|Texas Instruments Incorporated
| Programmable PCM Codec With Microphone Amps & Speaker Driver
| Marketing part#   Digital Voltage Range   Package-type   #pins
| TLV320A1110PBSRG4   2.7-3.3V   TQFP   32
| TLV320AIC1110PBS   2.7-3.3V   TQFP   32
| TLV320AIC1110PBSG4  2.7-3.3V   TQFP   32
| TLV320AIC1110PBSR   2.7-3.3V   TQFP   32
| TLV320AIC1110GQER   2.7-3.3V   BGA MICROSTAR JUNIOR   80
| TLV320AIC1110ZQER   2.7-3.3V   BGA MICROSTAR JUNIOR   80
[IBIS Ver]   3.2
[File name]   tlv320aic1110.ibs
|SIMDE Ver   V2.1 - 201006 - RHL4 - Build 390
[File Rev]   1.1
[Date]   10/06/2010
[Source]
| Texas Instruments Incorporated.
| Analog-eLab Design Center, HPA
| 12500 TI Blvd
| Dallas, TX -75243
| e-mail: elab_ibis@list.ti.com
| -Model generated from simulations in TISPICE
[Notes]   Revision History:
| Rev 1.0: 9/20/2010
| - Initial version of the model
| - Model generated from simulations in TISPICE
| - Model matched to SPICE simulation
| - C_comp although listed in numerical order of value are
|   obtained from varying PVT conditions. For PVT conditions for
|   each specific value refer the buffer description under
|   respective [Model]. IBIS model user is responsible for using
|   appropriate C_comp to simulate for Signal Integrity.
| Rev 1.1: 10/06/2010
| - io_open_drain_sda model VT table changed as per the review comments
[Disclaimer]
| This model is designed as an aid for customers of Texas Instruments.
| TI and its licensors and suppliers make no warranties, either expressed
| or implied, with respect to this  model, including the warranties of
| merchantability or fitness for a particular purpose. The model is
| provided solely on an "as is" basis. The entire risk as to its quality
| and performance is with the customer.
[Copyright]
 (C) Copyright 2010 Texas Instruments Incorporated.All rights reserved.
|   TLV320A1110PBSRG4/TLV320AIC1110PBS
[Component]   TLV320APBS
[Manufacturer]   TI
[Package]   |32 TQFP -  PBS package
|   typ   min   max
R_pkg   0.07184   0.06082   0.08808
L_pkg   2.28640nH   2.01650nH   2.68526nH
C_pkg   0.41135pF   0.38899pF   0.44791pF
[Pin]  signal_name   model_name   R_pin   L_pin   C_pin
1   MBIAS   TERM   0.08808   2.68526nH  0.41328pF
2   MIC1P   TERM   0.08391   2.54706nH  0.44791pF
3   MIC1N   TERM   0.07761   2.36771nH  0.42261pF
4   MIC2P   TERM   0.07618   2.30817nH  0.40996pF
5   MIC2N   TERM   0.07392   2.26536nH  0.40736pF
6   REXT   TERM   0.07368   2.29403nH  0.41316pF
7   MUXIN   TERM   0.07406   2.35917nH  0.43037pF
8   AVSS   GND   0.07533   2.44246nH  0.39927pF
9   MUXOUT1   TERM   0.07051   2.35058nH  0.39571pF
10   MUXOUT2   TERM   0.06517   2.18984nH  0.42182pF
11   SDA   io_opendrain_sda   0.06308   2.09272nH  0.40201pF
12   SCL   input_buffer   0.06082   2.01650nH  0.38966pF
13   DVDD   POWER   0.06336   2.06557nH  0.39394pF
14   DVSS   GND   0.06443   2.11869nH  0.40617pF
15   PCMI   input_buffer   0.06617   2.20906nH  0.42378pF
16   PCMO   tribuf_pcmo   0.07066   2.35247nH  0.39516pF
17   PCMCLK   input_pcmclk   0.07585   2.45373nH  0.39944pF
18   PCMSYN   input_buffer   0.07430   2.36520nH  0.42894pF
19   BUZZCON   tribuf_buzzcon   0.07499   2.32159nH  0.41275pF
20   PWRUPSEL   input_buffer   0.07407   2.26942nH  0.40286pF
21   _RESET   input_buffer   0.07381   2.26355nH  0.40434pF
22   MCLK   input_buffer   0.07436   2.30635nH  0.41540pF
23   VSS   GND   0.07577   2.38981nH  0.42966pF
24   PLLVSS   GND   0.08248   2.57901nH  0.40523pF
25   PLLVDD   POWER   0.07827   2.49816nH  0.40632pF
26   EARVSS   GND   0.07087   2.29522nH  0.43093pF
27   EAR1ON   TERM   0.06675   2.15760nH  0.40779pF
28   EARVDD   POWER   0.06793   2.14724nH  0.39773pF
29   EAR1OP   TERM   0.06150   2.02275nH  0.38899pF
30   EARVSS   GND   0.06028   2.03156nH  0.39750pF
31   EAR2O   TERM   0.06102   2.10259nH  0.41646pF
32   AVDD   POWER   0.06936   2.32089nH  0.39339pF
|   TLV320AIC1110GQER
[Component]   TLV320AIC1110GQER
[Manufacturer]   TI
[Package]   |80 BGA MICROSTAR JUNIOR - GQE package
|   typ   min   max
R_pkg   0.08490   0.06932   0.10116
L_pkg   1.58174nH   1.29375nH   1.88655nH
C_pkg   0.25756pF   0.23973pF   0.27588pF
[Pin]  signal_name   model_name   R_pin   L_pin   C_pin
A1   AVDD   POWER   0.09674  1.81151nH  0.23866pF
A2   EAR2O   TERM   0.08106  1.51327nH  0.25868pF
A3   EARVSS   GND   0.07517  1.40385nH  0.24777pF
A4   EAR1OP   TERM   0.07128  1.33092nH  0.24248pF
A5   EARVDD   POWER   0.07503  1.39865nH  0.24630pF
A6   EAR1ON   TERM   0.07460  1.38924nH  0.24697pF
A7   EARVSS   GND   0.08068  1.50050nH  0.25675pF
A8   PLLVDD   POWER   0.09065  1.68435nH  0.27183pF
A9   PLLVSS   GND   0.10018  1.86705nH  0.24341pF
B1   MBIAS   TERM   0.10116  1.88655nH  0.27588pF
B2   NC   NC   0.00000  0.00000nH  0.00000pF
B3   NC   NC   0.00000  0.00000nH  0.00000pF
B4   NC   NC   0.00000  0.00000nH  0.00000pF
B5   NC   NC   0.00000  0.00000nH  0.00000pF
B6   NC   NC   0.00000  0.00000nH  0.00000pF
B7   NC   NC   0.00000  0.00000nH  0.00000pF
B8   NC   NC   0.00000  0.00000nH  0.00000pF
B9   VSS   GND   0.09705  1.80167nH  0.27101pF
C1   MIC1P   TERM   0.09467  1.76610nH  0.27374pF
C2   NC   NC   0.00000  0.00000nH  0.00000pF
C4   NC   NC   0.00000  0.00000nH  0.00000pF
C5   NC   NC   0.00000  0.00000nH  0.00000pF
C6   NC   NC   0.00000  0.00000nH  0.00000pF
C7   NC   NC   0.00000  0.00000nH  0.00000pF
C8   NC   NC   0.00000  0.00000nH  0.00000pF
C9   MCLK   input_buffer   0.09113  1.69175nH  0.26699pF
D1   MIC1N   TERM   0.08667  1.61834nH  0.26258pF
D2   NC   NC   0.00000  0.00000nH  0.00000pF
D3   NC   NC   0.00000  0.00000nH  0.00000pF
D4   NC   NC   0.00000  0.00000nH  0.00000pF
D5   NC   NC   0.00000  0.00000nH  0.00000pF
D6   NC   NC   0.00000  0.00000nH  0.00000pF
D7   NC   NC   0.00000  0.00000nH  0.00000pF
D8   NC   NC   0.00000  0.00000nH  0.00000pF
D9   _RESET   input_buffer   0.08532  1.58372nH  0.25858pF
E1   MIC2P   TERM   0.08374  1.56425nH  0.25743pF
E2   NC   NC   0.00000  0.00000nH  0.00000pF
E3   NC   NC   0.00000  0.00000nH  0.00000pF
E4   NC   NC   0.00000  0.00000nH  0.00000pF
E5   NC   NC   0.00000  0.00000nH  0.00000pF
E6   NC   NC   0.00000  0.00000nH  0.00000pF
E7   NC   NC   0.00000  0.00000nH  0.00000pF
E8   NC   NC   0.00000  0.00000nH  0.00000pF
E9   PWRUPSEL   input_buffer   0.08338  1.54785nH  0.25370pF
F1   MIC2N   TERM   0.08482  1.58422nH  0.25973pF
F2   NC   NC   0.00000  0.00000nH  0.00000pF
F3   NC   NC   0.00000  0.00000nH  0.00000pF
F4   NC   NC   0.00000  0.00000nH  0.00000pF
F5   NC   NC   0.00000  0.00000nH  0.00000pF
F6   NC   NC   0.00000  0.00000nH  0.00000pF
F7   NC   NC   0.00000  0.00000nH  0.00000pF
F8   NC   NC   0.00000  0.00000nH  0.00000pF
F9   BUZZCON   tribuf_buzzcon   0.08449  1.56834nH  0.25426pF
G1   REXT   TERM   0.08858  1.65365nH  0.26206pF
G2   NC   NC   0.00000  0.00000nH  0.00000pF
G3   NC   NC   0.00000  0.00000nH  0.00000pF
G4   NC   NC   0.00000  0.00000nH  0.00000pF
G5   NC   NC   0.00000  0.00000nH  0.00000pF
G6   NC   NC   0.00000  0.00000nH  0.00000pF
G7   NC   NC   0.00000  0.00000nH  0.00000pF
G8   NC   NC   0.00000  0.00000nH  0.00000pF
G9   PCMSYN   input_buffer   0.08501  1.57820nH  0.25589pF
H1   MUXIN   TERM   0.09293  1.73427nH  0.27014pF
H2   NC   NC   0.00000  0.00000nH  0.00000pF
H3   NC   NC   0.00000  0.00000nH  0.00000pF
H4   NC   NC   0.00000  0.00000nH  0.00000pF
H5   NC   NC   0.00000  0.00000nH  0.00000pF
H6   NC   NC   0.00000  0.00000nH  0.00000pF
H7   NC   NC   0.00000  0.00000nH  0.00000pF
H8   NC   NC   0.00000  0.00000nH  0.00000pF
H9   PCMCLK   input_pcmclk   0.08868  1.64665nH  0.26211pF
J1   AVSS   GND   0.09974  1.86771nH  0.24131pF
J2   MUXOUT1   TERM   0.08328  1.55465nH  0.25850pF
J3   MUXOUT2   TERM   0.07537  1.40740nH  0.24832pF
J4   SDA   io_opendrain_sda   0.07152  1.33564nH  0.24231pF
J5   SCL   input_buffer   0.06932  1.29375nH  0.23973pF
J6   DVDD   POWER   0.07563  1.40832nH  0.24969pF
J7   DVSS   GND   0.08301  1.54355nH  0.26144pF
J8   PCMI   input_buffer   0.09030  1.67757nH  0.27218pF
J9   PCMO   tribuf_pcmo   0.10040  1.87191nH  0.24396pF
|   TLV320AIC1110ZQER
[Component]   TLV320AIC1110ZQER
[Manufacturer]   TI
[Package]   |80 BGA MICROSTAR JUNIOR - ZQE package
|   typ   min   max
R_pkg   0.08490   0.06932   0.10116
L_pkg   1.58174nH   1.29375nH   1.88655nH
C_pkg   0.25756pF   0.23973pF   0.27588pF
[Pin]  signal_name   model_name   R_pin   L_pin   C_pin
A1   AVDD   POWER   0.09674  1.81151nH  0.23866pF
A2   EAR2O   TERM   0.08106  1.51327nH  0.25868pF
A3   EARVSS   GND   0.07517  1.40385nH  0.24777pF
A4   EAR1OP   TERM   0.07128  1.33092nH  0.24248pF
A5   EARVDD   POWER   0.07503  1.39865nH  0.24630pF
A6   EAR1ON   TERM   0.07460  1.38924nH  0.24697pF
A7   EARVSS   GND   0.08068  1.50050nH  0.25675pF
A8   PLLVDD   POWER   0.09065  1.68435nH  0.27183pF
A9   PLLVSS   GND   0.10018  1.86705nH  0.24341pF
B1   MBIAS   TERM   0.10116  1.88655nH  0.27588pF
B2   NC   NC   0.00000  0.00000nH  0.00000pF
B3   NC   NC   0.00000  0.00000nH  0.00000pF
B4   NC   NC   0.00000  0.00000nH  0.00000pF
B5   NC   NC   0.00000  0.00000nH  0.00000pF
B6   NC   NC   0.00000  0.00000nH  0.00000pF
B7   NC   NC   0.00000  0.00000nH  0.00000pF
B8   NC   NC   0.00000  0.00000nH  0.00000pF
B9   VSS   GND   0.09705  1.80167nH  0.27101pF
C1   MIC1P   TERM   0.09467  1.76610nH  0.27374pF
C2   NC   NC   0.00000  0.00000nH  0.00000pF
C4   NC   NC   0.00000  0.00000nH  0.00000pF
C5   NC   NC   0.00000  0.00000nH  0.00000pF
C6   NC   NC   0.00000  0.00000nH  0.00000pF
C7   NC   NC   0.00000  0.00000nH  0.00000pF
C8   NC   NC   0.00000  0.00000nH  0.00000pF
C9   MCLK   input_buffer   0.09113  1.69175nH  0.26699pF
D1   MIC1N   TERM   0.08667  1.61834nH  0.26258pF
D2   NC   NC   0.00000  0.00000nH  0.00000pF
D3   NC   NC   0.00000  0.00000nH  0.00000pF
D4   NC   NC   0.00000  0.00000nH  0.00000pF
D5   NC   NC   0.00000  0.00000nH  0.00000pF
D6   NC   NC   0.00000  0.00000nH  0.00000pF
D7   NC   NC   0.00000  0.00000nH  0.00000pF
D8   NC   NC   0.00000  0.00000nH  0.00000pF
D9   _RESET   input_buffer   0.08532  1.58372nH  0.25858pF
E1   MIC2P   TERM   0.08374  1.56425nH  0.25743pF
E2   NC   NC   0.00000  0.00000nH  0.00000pF
E3   NC   NC   0.00000  0.00000nH  0.00000pF
E4   NC   NC   0.00000  0.00000nH  0.00000pF
E5   NC   NC   0.00000  0.00000nH  0.00000pF
E6   NC   NC   0.00000  0.00000nH  0.00000pF
E7   NC   NC   0.00000  0.00000nH  0.00000pF
E8   NC   NC   0.00000  0.00000nH  0.00000pF
E9   PWRUPSEL   input_buffer   0.08338  1.54785nH  0.25370pF
F1   MIC2N   TERM   0.08482  1.58422nH  0.25973pF
F2   NC   NC   0.00000  0.00000nH  0.00000pF
F3   NC   NC   0.00000  0.00000nH  0.00000pF
F4   NC   NC   0.00000  0.00000nH  0.00000pF
F5   NC   NC   0.00000  0.00000nH  0.00000pF
F6   NC   NC   0.00000  0.00000nH  0.00000pF
F7   NC   NC   0.00000  0.00000nH  0.00000pF
F8   NC   NC   0.00000  0.00000nH  0.00000pF
F9   BUZZCON   tribuf_buzzcon   0.08449  1.56834nH  0.25426pF
G1   REXT   TERM   0.08858  1.65365nH  0.26206pF
G2   NC   NC   0.00000  0.00000nH  0.00000pF
G3   NC   NC   0.00000  0.00000nH  0.00000pF
G4   NC   NC   0.00000  0.00000nH  0.00000pF
G5   NC   NC   0.00000  0.00000nH  0.00000pF
G6   NC   NC   0.00000  0.00000nH  0.00000pF
G7   NC   NC   0.00000  0.00000nH  0.00000pF
G8   NC   NC   0.00000  0.00000nH  0.00000pF
G9   PCMSYN   input_buffer   0.08501  1.57820nH  0.25589pF
H1   MUXIN   TERM   0.09293  1.73427nH  0.27014pF
H2   NC   NC   0.00000  0.00000nH  0.00000pF
H3   NC   NC   0.00000  0.00000nH  0.00000pF
H4   NC   NC   0.00000  0.00000nH  0.00000pF
H5   NC   NC   0.00000  0.00000nH  0.00000pF
H6   NC   NC   0.00000  0.00000nH  0.00000pF
H7   NC   NC   0.00000  0.00000nH  0.00000pF
H8   NC   NC   0.00000  0.00000nH  0.00000pF
H9   PCMCLK   input_pcmclk   0.08868  1.64665nH  0.26211pF
J1   AVSS   GND   0.09974  1.86771nH  0.24131pF
J2   MUXOUT1   TERM   0.08328  1.55465nH  0.25850pF
J3   MUXOUT2   TERM   0.07537  1.40740nH  0.24832pF
J4   SDA   io_opendrain_sda   0.07152  1.33564nH  0.24231pF
J5   SCL   input_buffer   0.06932  1.29375nH  0.23973pF
J6   DVDD   POWER   0.07563  1.40832nH  0.24969pF
J7   DVSS   GND   0.08301  1.54355nH  0.26144pF
J8   PCMI   input_buffer   0.09030  1.67757nH  0.27218pF
J9   PCMO   tribuf_pcmo   0.10040  1.87191nH  0.24396pF
[Model]  TERM
Model_type Terminator
C_comp   1.0e-20F  1.0e-20F  1.0e-20F
|   typ   min   max
[Voltage Range]   3.0V   2.7V   3.3V
[POWER Clamp Reference]   3.0V   2.7V   3.3V
[GND Clamp Reference]   0V   0V   0V
|Ambient Temperature   25   105   -40
|Junction Temperature
[Temperature Range]   65   125   -40
| Models and submodels in the file (6): input_buffer (Input), input_pcmclk (Input), tribuf_buzzcon (3-state), tribuf_pcmo (3-state), io_opendrain_sda (I/O_open_drain), TERM (Terminator)
